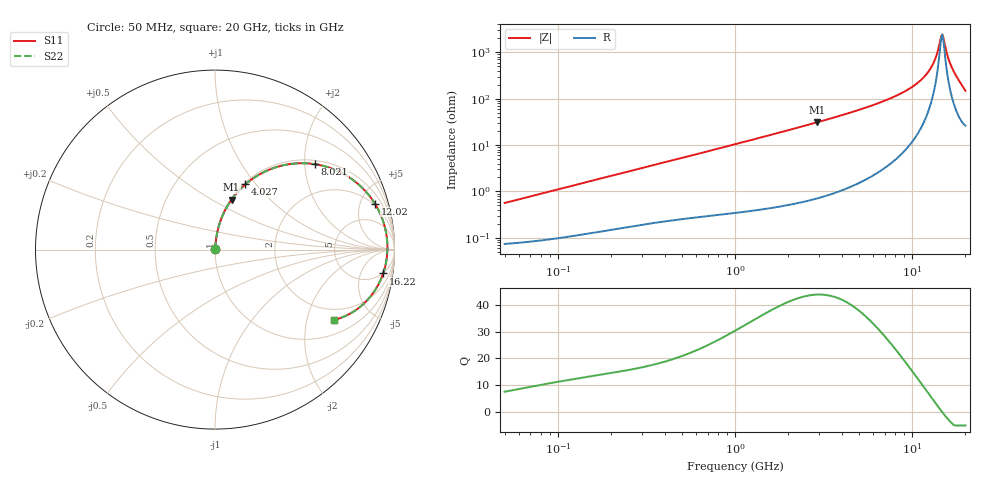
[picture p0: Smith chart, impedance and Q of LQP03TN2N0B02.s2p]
!Murata Part Number: LQP03TN2N0B02
!These Parameters are Measured in Series Mode Connection
!  o--[Z]--o
!Port1  Port2
!  o-------o
!Freq. Start=50[MHz] Stop=20[GHz], 401[Steps]
# Hz S RI R 50
!Freq.(Hz) S11(Real) S11(Imag) S21(Real) S21(Imag) S12(Real) S12(Imag) S22(Real) S22(Imag)
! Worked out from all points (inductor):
!   401 points, 50 MHz to 20 GHz, reference 50 ohm
!   read as one part in series: L = 1.77 nH near 51.52 MHz
!   highest Q = 43.8 at 2.896 GHz (marker M1), where L = 1.69 nH
!   self-resonance near 14.6 GHz
!   S11 on the Smith chart (normalised r, x): 50 MHz: 1.00, +0.01; 4.027 GHz: 1.02, +0.89; 8.021 GHz: 1.10, +2.25; 12.02 GHz: 1.81, +6.59; 16.22 GHz: 5, -12; 20 GHz: 1.52, -2.92
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5e7  0.00077 0.00558  0.9992 -0.00558  0.9992 -0.00558  0.00077 0.00558
1.364002e8  0.00139 0.0149  0.9986 -0.0149  0.9986 -0.0149  0.00139 0.0149
3.721004e8  0.00371 0.0392  0.9963 -0.0392  0.9963 -0.0392  0.00371 0.0392
1e9  0.014 0.1022  0.986 -0.1022  0.986 -0.1022  0.014 0.1022
2.728004e9  0.0822 0.2635  0.9178 -0.2635  0.9178 -0.2635  0.0822 0.2635
2.896447e9  0.0919 0.2778  0.9081 -0.2778  0.9081 -0.2778  0.0919 0.2778
4.026975e9  0.1698 0.3637  0.8302 -0.3637  0.8302 -0.3637  0.1698 0.3637
5.515528e9  0.3006 0.4446  0.6994 -0.4446  0.6994 -0.4446  0.3006 0.4446
7.442007e9  0.4973 0.4813  0.5027 -0.4813  0.5027 -0.4813  0.4973 0.4813
8.020766e9  0.5577 0.4759  0.4423 -0.4759  0.4423 -0.4759  0.5577 0.4759
1.019291e10  0.7648 0.3912  0.2352 -0.3912  0.2352 -0.3912  0.7648 0.3912
1.201863e10  0.8905 0.2566  0.1095 -0.2566  0.1095 -0.2566  0.8905 0.2566
1.276073e10  0.9242 0.1913  0.0758 -0.1913  0.0758 -0.1913  0.9242 0.1913
1.334722e10  0.9432 0.1371  0.0568 -0.1371  0.0568 -0.1371  0.9432 0.1371
1.438523e10  0.9599 0.0386  0.0401 -0.0386  0.0401 -0.0386  0.9599 0.0386
1.460232e10  0.9607 0.0178  0.0393 -0.0178  0.0393 -0.0178  0.9607 0.0178
1.482269e10  0.9605 -0.00316  0.0395 0.00316  0.0395 0.00316  0.9605 -0.00316
1.504638e10  0.9593 -0.0244  0.0407 0.0244  0.0407 0.0244  0.9593 -0.0244
1.621653e10  0.937 -0.1327  0.063 0.1327  0.063 0.1327  0.937 -0.1327
1.696185e10  0.9086 -0.1977  0.0914 0.1977  0.0914 0.1977  0.9086 -0.1977
1.774144e10  0.8667 -0.2608  0.1333 0.2608  0.1333 0.2608  0.8667 -0.2608
2e10  0.6609 -0.3919  0.3391 0.3919  0.3391 0.3919  0.6609 -0.3919
